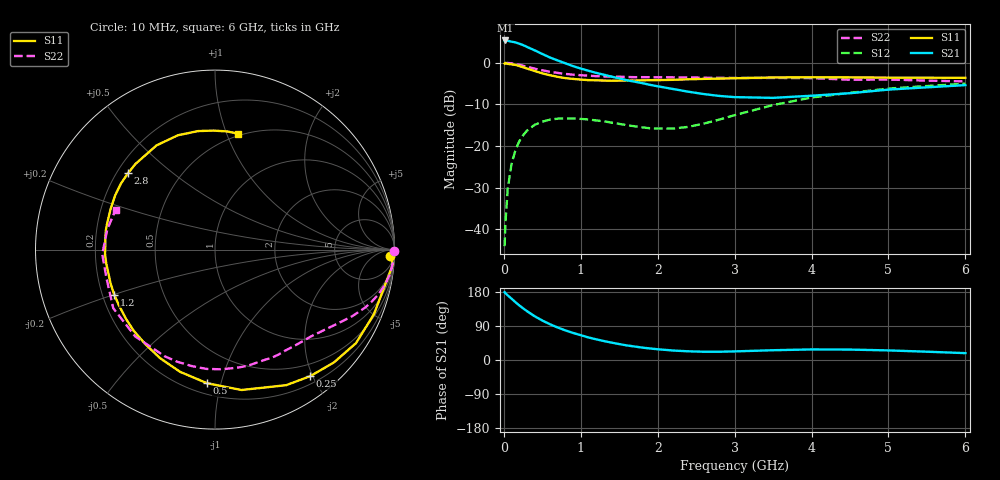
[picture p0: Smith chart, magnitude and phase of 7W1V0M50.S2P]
! Infineon Technologies  Discrete & RF Semiconductors
! BFS17W
! Si NPN RF Bipolar Junction Transistor in SOT323
! VCE = 1 V  IC = 0.5 mA
! Common Emitter S-Parameters:  August  1999
# GHz  S  MA  R  50
!  f  S11  S21  S12  S22
! GHz  MAG  ANG  MAG  ANG  MAG  ANG  MAG  ANG
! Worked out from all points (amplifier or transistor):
!   36 points, 10 MHz to 6 GHz, reference 50 ohm
!   highest |S21| = 5.3 dB at 20 MHz (marker M1)
!   |S21| within 3 dB of that: start of sweep to 472.2 MHz
!   unconditionally stable (mu >= 1): 1.095 GHz to end of sweep
!   at 250 MHz: K = 0.26, MSG = 10.8 dB, |S12| = -17.4 dB
!   at 1.4 GHz: K = 1.25, MAG = 2.5 dB, |S12| = -14.4 dB
!   at 6 GHz: K = 1.13, MAG = -2.4 dB, |S12| = -5.0 dB
!   S11 on the Smith chart (normalised r, x): 10 MHz: 25, -39; 250 MHz: 0.31, -1.96; 500 MHz: 0.27, -0.91; 1.2 GHz: 0.25, -0.20; 2.8 GHz: 0.24, +0.36; 6 GHz: 0.48, +1.10
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0.01  0.9772 -2.1  1.836 179.0  0.0063 87.6  0.9999 -0.3
0.02  0.9938 -4.8  1.851 176.4  0.0116 87.5  0.9887 -1.5
0.05  0.969 -11.3  1.837 170.7  0.0307 83.7  0.994 -4.1
0.1  0.956 -22.1  1.79 161.9  0.0608 76.1  0.9841 -8.1
0.15  0.9426 -33.6  1.756 152.7  0.0892 69.0  0.9661 -11.8
0.25  0.8823 -53.1  1.629 136.4  0.1348 57.1  0.9199 -18.4
0.3  0.8531 -62.3  1.55 129.0  0.1527 52.2  0.8969 -21.1
0.4  0.7961 -79.3  1.41 115.5  0.1799 43.1  0.85 -25.9
0.5  0.7458 -93.4  1.274 104.2  0.1961 36.0  0.8108 -29.7
0.6  0.7081 -106.0  1.156 94.3  0.2079 30.1  0.7797 -33.2
0.8  0.6539 -126.6  0.985 78.1  0.2151 22.0  0.7348 -39.6
1.1  0.6186 -149.9  0.802 59.5  0.2086 14.7  0.6993 -48.9
1.2  0.6151 -156.0  0.756 54.6  0.2032 13.2  0.6907 -52.3
1.6  0.6133 -177.8  0.616 38.4  0.1783 13.3  0.6742 -65.6
2.2  0.6243 158.6  0.484 25.0  0.1625 30.4  0.668 -86.9
2.8  0.6451 138.7  0.4 21.8  0.2077 47.9  0.6591 -108.7
3.5  0.6658 119.3  0.379 25.8  0.3109 50.4  0.657 -132.6
4  0.6697 108.0  0.402 27.9  0.3825 45.5  0.6542 -150.1
4.5  0.6671 98.2  0.431 27.5  0.4356 39.4  0.625 -165.4
5  0.6632 90.7  0.476 25.3  0.4896 33.6  0.6287 -177.7
5.5  0.6617 84.2  0.507 21.9  0.5259 27.8  0.6104 169.3
6  0.6587 78.9  0.539 18.1  0.5608 22.3  0.5969 158.2
